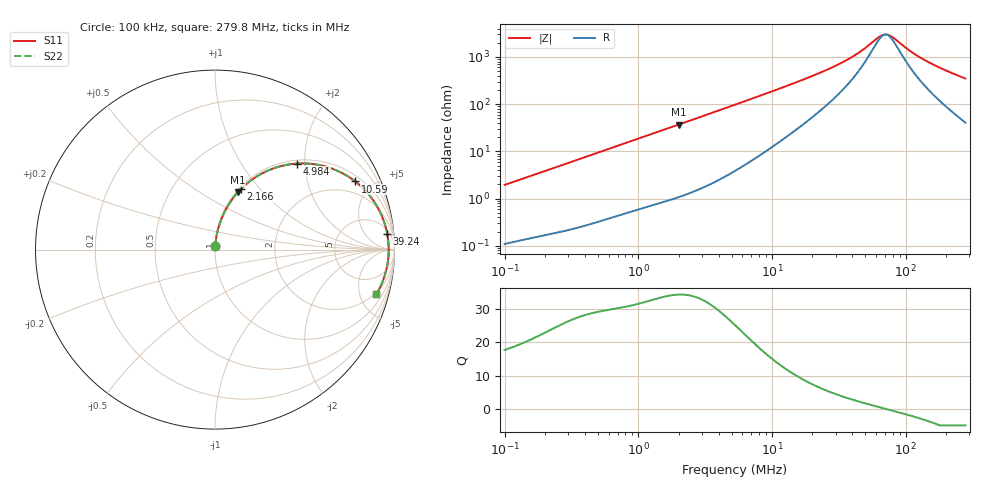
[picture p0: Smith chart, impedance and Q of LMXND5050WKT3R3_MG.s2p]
! LMXND5050WKT3R3_MG  S-PARAMETER MODEL  ( General Type )
! Model Generated by TAIYO YUDEN Corporation (https://www.yuden.co.jp/en/)
! Version 1.0
! TAIYO YUDEN Control No. 191023NI43SB-FBB
! Copyright(c) 2019 TAIYO YUDEN CO.,LTD. All Rights Reserved.
! Product Description (link to TY-COMPAS)
! https://ds.yuden.co.jp/TYCOMPAS/or/detail?pn=LMXND5050WKT3R3NMG&u=M
! Products Name : Inductors
! Characteristics :
!  Inductance : 3.3 uH , SRF(min) : 46 MHz , DC Resistance(max) : 0.0576 Ohm
!  Rated Current : Saturation :2400 mA , Temp Rise : 2400 mA (40 degC)
!  Case Size : 4.9 x 4.9 / 0.193 x 0.193 [mm/inch] , Thickness : 2 / 0.079 [mm/inch]
!  (Conditions: Temperature = 25 degC , DC Bias Current/Voltage = 0A / 0V)
! External Node Assignments :
!  1  o---GGG---o  2
! GND o---------o GND
! Frequency Range : 0.1MHz  -  279.750408MHz  [ 402 STEP ]
# MHz S RI R 50
! Freq[MHz].  S11 Real  S11 Imag  S21 Real  S21 Imag  S12 Real  S12 Imag  S22 Real  S22 Imag
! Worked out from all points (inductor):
!   401 points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, 100 kHz to 279.8 MHz, reference 50 ohm
!   read as one part in series: L = 3.08 uH near 104 kHz
!   highest Q = 34.4 at 2.001 MHz (marker M1), where L = 2.93 uH
!   self-resonance near 70.84 MHz
!   S11 on the Smith chart (normalised r, x): 100 kHz: 1.00, +0.04; 2.166 MHz: 1.02, +0.80; 4.984 MHz: 1.07, +1.84; 10.59 MHz: 1.28, +3.95; 39.24 MHz: 7, +19; 279.8 MHz: 1.81, -6.93
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0.1  0.00148 0.0195  0.9985 -0.0195  0.9985 -0.0195  0.00148 0.0195
0.377863  0.00761 0.0708  0.9924 -0.0708  0.9924 -0.0708  0.00761 0.0708
0.771869  0.0248 0.1401  0.9752 -0.1401  0.9752 -0.1401  0.0248 0.1401
1.427803  0.0716 0.2434  0.9284 -0.2434  0.9284 -0.2434  0.0716 0.2434
2.00058  0.1269 0.3187  0.8731 -0.3187  0.8731 -0.3187  0.1269 0.3187
2.165826  0.1446 0.3375  0.8554 -0.3375  0.8554 -0.3375  0.1446 0.3375
3.220788  0.2664 0.4269  0.7336 -0.4269  0.7336 -0.4269  0.2664 0.4269
4.983501  0.4592 0.4796  0.5408 -0.4796  0.5408 -0.4796  0.4592 0.4796
5.289144  0.488 0.4804  0.512 -0.4804  0.512 -0.4804  0.488 0.4804
7.265344  0.6375 0.4563  0.3625 -0.4563  0.3625 -0.4563  0.6375 0.4563
10.592  0.7813 0.3799  0.2187 -0.3799  0.2187 -0.3799  0.7813 0.3799
19.9857  0.9134 0.2219  0.0866 -0.2219  0.0866 -0.2219  0.9134 0.2219
29.13675  0.9461 0.1424  0.0539 -0.1424  0.0539 -0.1424  0.9461 0.1424
39.23693  0.9593 0.0894  0.0407 -0.0894  0.0407 -0.0894  0.9593 0.0894
47.84805  0.9642 0.0578  0.0358 -0.0578  0.0358 -0.0578  0.9642 0.0578
64.43445  0.9675 0.0137  0.0325 -0.0137  0.0325 -0.0137  0.9675 0.0137
69.75669  0.9677 0.00222  0.0323 -0.00222  0.0323 -0.00222  0.9677 0.00222
75.51853  0.9676 -0.00923  0.0324 0.00923  0.0324 0.00923  0.9676 -0.00923
110.0969  0.9633 -0.0654  0.0367 0.0654  0.0367 0.0654  0.9633 -0.0654
136.9498  0.9571 -0.101  0.0429 0.101  0.0429 0.101  0.9571 -0.101
191.8886  0.9392 -0.1637  0.0608 0.1637  0.0608 0.1637  0.9392 -0.1637
279.7504  0.8995 -0.2477  0.1005 0.2477  0.1005 0.2477  0.8995 -0.2477
